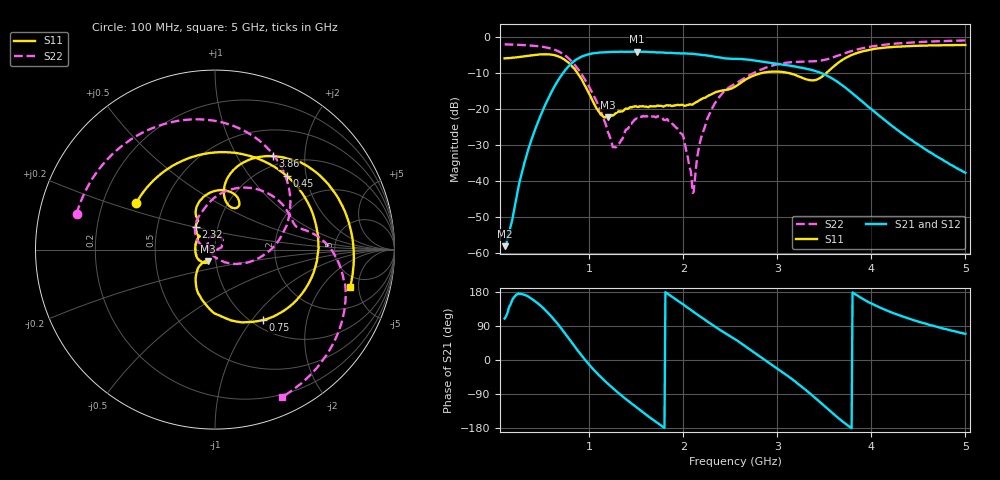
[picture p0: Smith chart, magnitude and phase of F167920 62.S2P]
!  2-Port S-parameters saved by WinCal
! VAR MeasName=S-Parameters (CALIBRATED_DATA) read from VNA (N5242A)
! VAR MeasDate=2016-11-22 9:58:37
! VAR NAME=F167920 62
! VAR FILENAME=F167920 62.S2P
! VAR DATE=2016-11-22 9:58:37
! VAR PHYS_PORTS=1,2
# Hz S DB R 50
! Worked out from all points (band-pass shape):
!   491 points, 100 MHz to 5 GHz, reference 50 ohm
!   highest |S21| = -3.99 dB at 1.51 GHz (marker M1); lowest = -58.0 dB at 100 MHz (marker M2)
!   |S21| within 3 dB of the highest: 824 MHz to 2.895 GHz (2.071 GHz wide, 111 % of centre)
!   lowest |S11| = -22.3 dB at 1.2 GHz (marker M3), VSWR 1.17, Z = 45.6 - j5.95 ohm
!   |S11| at or under -10 dB: 874.7 MHz to 2.825 GHz (1.95 GHz wide, 105 % of centre); 3.133 GHz to 3.518 GHz (385.3 MHz wide, 11.6 % of centre)
!   |S22| runs from -43.2 to -0.9 dB; largest |S21 - S12| = 0.00097
!   S11 on the Smith chart (normalised r, x): 100 MHz: 0.35, +0.24; 450 MHz: 1.28, +1.56; 750 MHz: 1.12, -1.14; 2.32 GHz: 0.78, +0.20; 3.86 GHz: 0.86, +1.42; 5 GHz: 3.72, -3.99
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1e8  -5.86 149.4  -57.97 109.4  -58.19 105.6  -1.98 165.5
2.9e8  -5.37 93.1  -36.93 173.5  -36.93 173.4  -2.15 137.0
4.5e8  -4.83 45.4  -23.86 150.0  -23.86 150.1  -2.47 110.1
6e8  -4.84 -2.8  -15.13 114.1  -15.13 114.2  -3.20 79.8
7.5e8  -6.46 -55.6  -8.96 67.7  -8.95 67.8  -5.18 42.8
9.2e8  -11.69 -111.2  -5.36 11.7  -5.35 11.7  -10.36 -1.3
1.04e9  -17.87 -133.4  -4.47 -23.8  -4.48 -23.8  -15.78 -28.5
1.2e9  -22.26 -122.8  -4.09 -63.2  -4.09 -63.3  -26.43 -78.7
1.28e9  -21.12 -122.9  -4.06 -80.7  -4.06 -80.6  -30.53 -145.9
1.51e9  -19.30 -162.7  -3.99 -126.3  -3.99 -126.3  -22.57 108.8
1.74e9  -19.07 163.4  -4.20 -168.5  -4.20 -168.6  -21.98 70.8
1.99e9  -18.74 140.4  -4.48 148.3  -4.48 148.3  -26.98 29.6
2.11e9  -18.45 140.3  -4.63 126.8  -4.63 126.7  -43.01 -118.9
2.19e9  -17.22 137.8  -4.89 112.9  -4.89 112.9  -27.87 176.3
2.32e9  -15.57 130.2  -5.32 90.7  -5.32 90.6  -19.08 152.0
2.55e9  -13.75 119.8  -5.97 55.2  -5.98 55.2  -12.93 108.1
2.91e9  -9.61 86.6  -7.04 -7.0  -7.05 -7.1  -8.16 61.9
3.37e9  -11.96 67.6  -9.10 -93.1  -9.10 -93.1  -6.69 18.4
3.6e9  -8.10 80.6  -11.70 -143.0  -11.71 -143.0  -5.53 11.2
3.86e9  -4.27 58.3  -16.90 168.5  -16.92 168.5  -3.33 -4.5
4.19e9  -2.77 30.6  -23.99 128.0  -24.01 128.2  -1.92 -26.6
5e9  -2.14 -15.5  -37.59 69.4  -37.63 69.3  -0.89 -65.8
